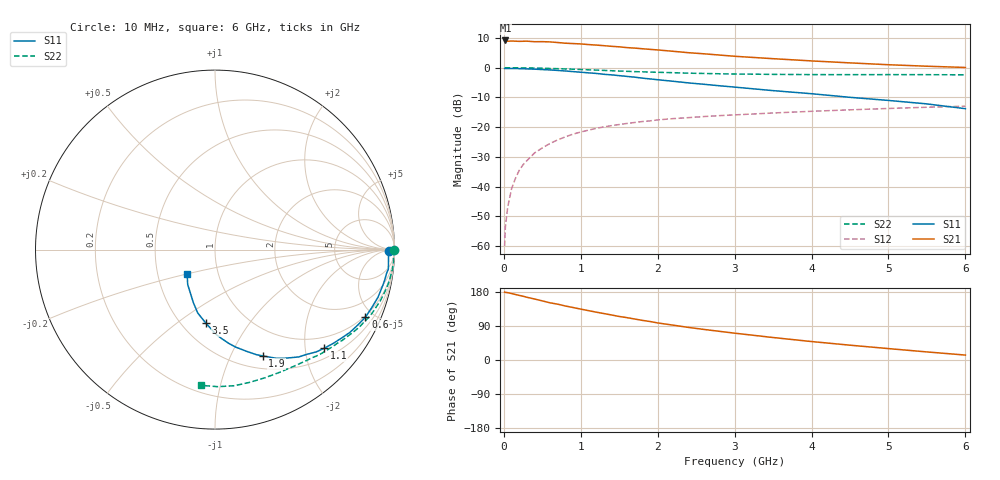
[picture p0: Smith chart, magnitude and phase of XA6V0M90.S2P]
! SIEMENS Discrete & RF Semiconductors
! BFY180
! Si NPN RF Bipolar Junction Transistor in MICRO-X
! VCE = 6 V  IC = 0.9 mA
! Common Emitter S-Parameters:  May  1997
# GHz  S  MA  R  50
!  f  S11  S21  S12  S22
! GHz  MAG  ANG  MAG  ANG  MAG  ANG  MAG  ANG
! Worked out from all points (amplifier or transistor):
!   36 points, 10 MHz to 6 GHz, reference 50 ohm
!   highest |S21| = 9.2 dB at 20 MHz (marker M1)
!   |S21| within 3 dB of that: start of sweep to 1.903 GHz
!   unconditionally stable (mu >= 1): 4.379 GHz to end of sweep
!   at 250 MHz: K = 0.08, MSG = 20.8 dB, |S12| = -32.6 dB
!   at 1.4 GHz: K = 0.46, MSG = 13.3 dB, |S12| = -19.5 dB
!   at 6 GHz: K = 1.04, MAG = 5.3 dB, |S12| = -12.9 dB
!   S11 on the Smith chart (normalised r, x): 10 MHz: 62, -10; 600 MHz: 0.93, -4.48; 1.1 GHz: 0.72, -2.42; 1.9 GHz: 0.65, -1.33; 3.5 GHz: 0.65, -0.64; 6 GHz: 0.71, -0.20
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0.01  0.969 -0.3  2.822 179.3  0.001 79.7  0.9978 -0.1
0.02  0.9681 -0.7  2.874 178.5  0.0021 94.5  0.9999 -0.5
0.05  0.9675 -2.1  2.789 177.7  0.0045 86.1  0.9984 -1.3
0.1  0.9688 -4.0  2.814 175.4  0.0092 89.1  0.9953 -2.6
0.2  0.9647 -8.0  2.777 170.5  0.0188 85.2  0.9955 -5.1
0.3  0.9559 -12.1  2.796 165.5  0.0274 81.6  0.9909 -7.7
0.4  0.9462 -16.3  2.737 160.9  0.037 78.4  0.9869 -10.1
0.5  0.9315 -20.3  2.744 156.0  0.0449 75.8  0.9798 -12.6
0.6  0.9188 -24.2  2.717 150.9  0.0533 72.6  0.9712 -15.0
1  0.8405 -38.5  2.513 134.3  0.083 62.2  0.9343 -24.1
1.1  0.8204 -42.0  2.451 130.3  0.0893 60.0  0.9225 -26.1
1.2  0.8019 -45.3  2.404 126.3  0.0955 57.5  0.9129 -28.2
1.5  0.7361 -54.9  2.245 114.9  0.1109 51.5  0.8796 -33.8
1.9  0.6488 -65.9  2.036 101.6  0.1277 45.0  0.8447 -40.5
2.2  0.5922 -72.9  1.889 92.0  0.1394 40.6  0.8253 -45.2
2.4  0.5556 -78.0  1.789 86.0  0.1448 38.3  0.8101 -48.0
2.8  0.4979 -85.6  1.635 75.7  0.1565 34.0  0.7916 -53.3
3.5  0.4121 -97.2  1.419 59.3  0.1734 27.6  0.7728 -62.2
4  0.3657 -105.3  1.302 48.7  0.1851 23.3  0.7665 -68.5
4.5  0.318 -112.4  1.206 39.1  0.1959 19.3  0.7645 -75.1
5.5  0.2466 -128.1  1.06 21.3  0.2166 11.3  0.7639 -88.8
6  0.2049 -139.3  1.01 13.0  0.2257 7.1  0.7604 -95.7
